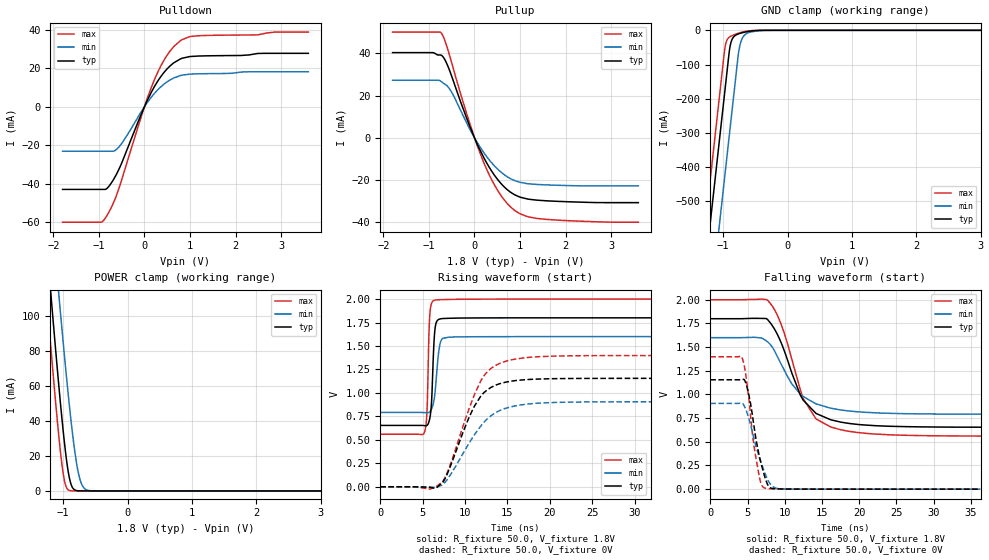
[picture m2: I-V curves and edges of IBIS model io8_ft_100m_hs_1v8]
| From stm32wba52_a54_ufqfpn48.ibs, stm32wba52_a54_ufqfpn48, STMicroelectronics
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[Model]   io8_ft_100m_hs_1v8
Model_type I/O
Polarity   Non-Inverting
Enable   Active-Low
| CAP_THRESHOLD on pad IOFT is "UDTCAPC" :
| Rising=30.0% of vddiom   Falling=70.0% of vddiom
| C_comp min and max val. don't necessarily correlate with the min and max pvt
| but are the smallest and greatest pad capacitance found.
| var   typ   min   max
C_comp   2.20760pF  2.09930pF  2.39591pF
|C_comp_pullup   1.38215pF  1.31805pF  1.46447pF
|C_comp_pulldown   825.44519fF  781.25002fF  931.44109fF
Vinl = 800.0mV
Vinh = 1.0V
Vmeas = 900.0mV   | Reference voltage for timing measurements
Cref  = 50.0pF   | Timing specification test load capacitance value
Rref  = 1.0MOhm   | Timing specification test load resistance value
Vref  = 990.0mV   | Timing specification test load voltage
[Model Spec]
| TIME_THRESHOLD on pin ZIV11 is "CMOS" :
| Rising=50.0% of vdd   Falling=50.0% of vdd
Vinl 702.50000mV 642.50000mV 771.50000mV
Vinh 1.09050V 944.50000mV 1.21950V
| variable   typ   min   max
[Temperature Range] 25.0 140.0 -40.0
| variable   typ   min   max
[Voltage Range] 1.8V 1.6V 2.0V
| variable   typ   min   max
[POWER Clamp Reference] 1.8V 1.6V 2.0V
| variable   typ   min   max
[GND Clamp Reference] 0V 0V 0V
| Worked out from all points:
|   slope of the pulldown table from 0 to 0.27 V, typ, clamps not added: 21.7 ohm
|   slope of the pullup table from 0 to 0.27 V, typ, clamps not added: 22.5 ohm
|   GND clamp passes 1 mA (typ) near -0.51 V on its own axis
|   POWER clamp passes 1 mA (typ) near -0.83 V on its own axis
|   rising waveform, R_fixture 50.0, V_fixture 1.8V: 20-80 % time 322ps typ, 506ps min, 248ps max; typ from 0.654 V to 1.8 V
|   falling waveform, R_fixture 50.0, V_fixture 1.8V: 20-80 % time 3.79ns typ, 4.25ns min, 3.69ns max; typ from 1.8 V to 0.654 V
|   rising waveform, R_fixture 50.0, V_fixture 0V: 20-80 % time 3.24ns typ, 3.99ns min, 3.37ns max; typ from 0 V to 1.16 V
|   falling waveform, R_fixture 50.0, V_fixture 0V: 20-80 % time 1.6ns typ, 2.02ns min, 1.33ns max; typ from 1.16 V to 0 V
[POWER Clamp]
-1.8V     396.4mA    438.1mA    365.5mA
-1.26V    143.5mA    194.6mA    112.6mA
-1.19V    112.3mA    164.2mA    81.56mA
-1.06V    57.23mA    109.3mA    28.68mA
-1.02V    41.75mA    93.06mA    15.5mA
-980mV    27.6mA     77.28mA    5.935mA
-910mV    8.693mA    51.24mA    382.3uA
-850mV    1.642mA    31.41mA    23.97uA
-760mV    69.41uA    9.714mA    358.6nA
-700mV    7.83uA     2.919mA    21.79nA
-620mV    424.6nA    410.3uA    573.9pA
3.6V      0A         0A         0A
[GND Clamp]
-1.8V     -1.583A    -1.83A     -1.456A
-1.43V    -953.9mA   -1.201A    -826.8mA
-1.24V    -630.9mA   -877.8mA   -503.8mA
-1.05V    -307.9mA   -554.8mA   -180.8mA
-970mV    -171.9mA   -418.8mA   -48.31mA
-910mV    -69.87mA   -316.8mA   -20.91mA
-880mV    -36.5mA    -265.8mA   -17.19mA
-830mV    -17.68mA   -180.8mA   -12.97mA
-750mV    -9.66mA    -53.66mA   -7.697mA
-690mV    -6.479mA   -19.19mA   -4.622mA
-600mV    -3.058mA   -6.478mA   -1.59mA
3.6V      1.281nA    1.39uA     517.2pA
| variable   typ   min   max
[Pullup Reference] 1.8V 1.6V 2.0V
| variable   typ   min   max
[Pulldown Reference] 0V 0V 0V
[Pullup]
-1.8V     40.39mA    27.3mA     50.13mA
-910mV    40.38mA    27.3mA     50.13mA
-720mV    39.03mA    26.51mA    49.35mA
-630mV    36.17mA    25.17mA    44.85mA
-510mV    29.75mA    21.9mA     36.26mA
-120mV    6.338mA    4.782mA    7.854mA
190mV     -8.788mA   -6.58mA    -11.01mA
530mV     -20.35mA   -15.28mA   -25.66mA
880mV     -26.99mA   -20.26mA   -34.39mA
1.18V     -29.09mA   -21.8mA    -37.49mA
1.56V     -29.85mA   -22.32mA   -38.64mA
3.6V      -30.74mA   -22.8mA    -40.02mA
[Pulldown]
-1.8V     -42.97mA   -23.15mA   -59.99mA
-950mV    -42.97mA   -23.15mA   -59.99mA
-850mV    -42.87mA   -23.15mA   -57.45mA
-670mV    -37.41mA   -23.03mA   -49.3mA
-550mV    -31.91mA   -20.61mA   -41.6mA
10mV      539.8uA    356.7uA    722uA
230mV     10.88mA    7.174mA    14.64mA
500mV     19.69mA    12.93mA    26.79mA
790mV     24.78mA    16.15mA    34.26mA
1V        26.02mA    16.89mA    36.38mA
1.18V     26.27mA    17.05mA    36.82mA
3.6V      27.68mA    18.11mA    38.71mA
[Ramp]
dV/dt_r 693.10642mV/3.20069ns 543.2599mV/3.98937ns 838.8394mV/3.36495ns
dV/dt_f 687.69176mV/3.59133ns 484.93668mV/4.15982ns 864.00325mV/3.42448ns
R_load = 50.0
| Removed startup time: 0s 0s 0s  .
| Removed end time: 36.25ns.
[Rising Waveform]
R_fixture   = 50.0
V_fixture   = 1.8V
V_fixture_min = 1.6V
V_fixture_max = 2.0V
0s        653.8mV    791.8mV    560mV
5.2ns     651.3mV    790.6mV    578.8mV
5.5ns     653.3mV    788.2mV    782.7mV
5.75ns    694.7mV    792.7mV    1.649V
5.85ns    732.3mV    799.6mV    1.84V
6.05ns    902.5mV    828.1mV    1.955V
6.35ns    1.561V     928.9mV    1.986V
6.95ns    1.785V     1.473V     1.993V
7.4ns     1.793V     1.582V     1.994V
36.25ns   1.8V       1.6V       2V
| Removed startup time: 0s 0s 0s  .
| Removed end time: 99.25ns.
[Falling Waveform]
R_fixture   = 50.0
V_fixture   = 1.8V
V_fixture_min = 1.6V
V_fixture_max = 2.0V
0s        1.8V       1.6V       2V
6.1ns     1.804V     1.603V     2.004V
7.7ns     1.791V     1.556V     1.994V
9.65ns    1.52V      1.3V       1.711V
10.95ns   1.226V     1.112V     1.371V
12.5ns    938.4mV    976.9mV    951.9mV
14.2ns    799.7mV    900.8mV    741.2mV
18.15ns   699.8mV    830.1mV    617.1mV
32.4ns    655.1mV    793mV      562mV
99.25ns   653.8mV    791.8mV    560mV
| Removed startup time: 0s 0s 0s  .
| Removed end time: 99.2ns.
[Rising Waveform]
R_fixture   = 50.0
V_fixture   = 0V
V_fixture_min = 0V
V_fixture_max = 0V
0s        4.66nV     680.4nV    3.931nV
5.85ns    -5.884mV   -3.215mV   -25.55mV
7.35ns    44.72mV    20.3mV     53.69mV
8.1ns     178.5mV    103.1mV    195.5mV
10.4ns    722.8mV    453mV      812.7mV
11.95ns   975.3mV    657.2mV    1.142V
13.45ns   1.076V     780.8mV    1.285V
16ns      1.132V     862.8mV    1.362V
24.3ns    1.154V     903.7mV    1.397V
99.2ns    1.155V     905.4mV    1.398V
| Removed startup time: 0s 0s 0s  .
| Removed end time: 36.25ns.
[Falling Waveform]
R_fixture   = 50.0
V_fixture   = 0V
V_fixture_min = 0V
V_fixture_max = 0V
0s        1.155V     905.5mV    1.398V
4.25ns    1.155V     908.9mV    1.392V
5.05ns    1.041V     780.2mV    1.032V
5.7ns     756.5mV    588.3mV    556.6mV
6.15ns    521.1mV    448.7mV    320.3mV
6.7ns     310.8mV    306.2mV    90.41mV
7.15ns    175.4mV    208.3mV    18.12mV
8ns       17.52mV    60.91mV    4.816mV
9.65ns    1.901mV    2.272mV    1.585mV
36.25ns   26.78nV    1.164uV    2.242uV
